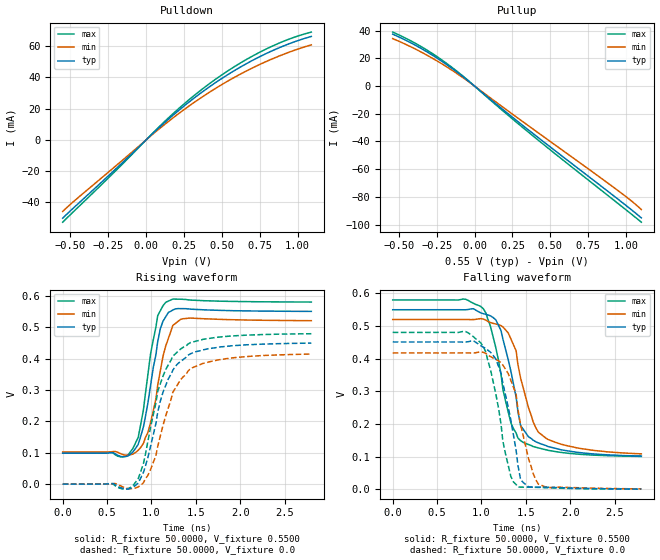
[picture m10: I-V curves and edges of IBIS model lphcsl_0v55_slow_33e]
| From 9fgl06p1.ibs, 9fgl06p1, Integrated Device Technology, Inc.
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[Model]   lphcsl_0v55_slow_33e
Model_type Output
Polarity   Inverting
Enable   Active-High
Vmeas =  0.4000V
Cref =   2.0000pF
Rref =   0.0
Vref =   0.4000V
C_comp   1.1000pF   1.0000pF   1.2000pF
[Temperature Range]   25.0000   85.0000   -40.0
[Voltage Range]   0.5500V   0.5200V   0.5800V
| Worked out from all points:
|   slope of the pulldown table from 0 to 0.083 V, typ, clamps not added: 10.9 ohm
|   slope of the pullup table from 0 to 0.083 V, typ, clamps not added: 10.9 ohm
|   rising waveform, R_fixture 50.0000, V_fixture 0.5500: 20-80 % time 160ps typ, 177ps min, 156ps max; typ from 0.099 V to 0.55 V
|   rising waveform, R_fixture 50.0000, V_fixture 0.0: 20-80 % time 271ps typ, 286ps min, 264ps max; typ from 0 V to 0.449 V
|   falling waveform, R_fixture 50.0000, V_fixture 0.5500: 20-80 % time 210ps typ, 239ps min, 228ps max; typ from 0.55 V to 0.102 V
|   falling waveform, R_fixture 50.0000, V_fixture 0.0: 20-80 % time 190ps typ, 211ps min, 199ps max; typ from 0.451 V to 0.001 V
[Pulldown]
|Voltage   I(typ)   I(min)   I(max)
-550mV    -50.08mA   -45.78mA   -52.65mA
-470mV    -42.74mA   -38.74mA   -45.07mA
-210mV    -19.46mA   -17.46mA   -20.63mA
130mV     11.78mA    10.51mA    12.52mA
250mV     21.68mA    19.4mA     23.02mA
390mV     32.07mA    28.79mA    33.99mA
570mV     43.66mA    39.38mA    46.13mA
750mV     53.32mA    48.34mA    56.16mA
930mV     61.07mA    55.69mA    64.05mA
1.09V     66.25mA    60.88mA    69.05mA
[Pullup]
|Voltage   I(typ)   I(min)   I(max)
-540mV    37.52mA    34.32mA    39.03mA
-440mV    32.37mA    29.43mA    33.82mA
-340mV    26.43mA    23.9mA     27.73mA
-240mV    19.68mA    17.7mA     20.72mA
-140mV    12.09mA    10.82mA    12.77mA
360mV     -32.05mA   -29mA      -33.69mA
920mV     -79.46mA   -73.36mA   -82.52mA
1.02V     -88.05mA   -81.67mA   -91.22mA
1.1V      -95.23mA   -89.17mA   -98.31mA
[Ramp]
| variable   typ   min   max
dV/dt_r  0.2696/0.2691n   0.2487/0.2857n   0.2876/0.2561n
dV/dt_f  0.2689/0.2333n   0.2469/0.2701n   0.2876/0.2220n
R_load = 50.0000
[Rising Waveform]
R_fixture= 50.0000
V_fixture= 0.5500
V_fixture_min= 0.5200
V_fixture_max= 0.5800
|time   V(typ)   V(min)   V(max)
0s        98.56mV    102.4mV    98.79mV
680ps     87.06mV    93.93mV    86.97mV
790ps     101.9mV    95.69mV    113.2mV
850ps     126.6mV    107.7mV    148.9mV
960ps     259.3mV    164.8mV    350.4mV
1.07ns    454.4mV    315.3mV    537.1mV
1.16ns    533.3mV    439.9mV    579.4mV
1.24ns    554.9mV    505.8mV    589.8mV
1.36ns    559.2mV    527.3mV    588.9mV
2.8ns     550.5mV    520.9mV    580.3mV
[Rising Waveform]
R_fixture= 50.0000
V_fixture= 0.0
V_fixture_min= 0.0
V_fixture_max= 0.0
|time   V(typ)   V(min)   V(max)
0s        0V         0V         0V
790ps     -10.68mV   -14.72mV   -5.101mV
910ps     37.96mV    4.791mV    66.39mV
1.05ns    193.4mV    91.13mV    259.1mV
1.07ns    229.3mV    119.9mV    295.8mV
1.13ns    293.2mV    187.7mV    344.4mV
1.24ns    362.9mV    292.5mV    407.7mV
1.44ns    415.6mV    368.5mV    451.3mV
1.89ns    440.5mV    401.6mV    471.9mV
2.8ns     449.4mV    414.5mV    479.3mV
[Falling Waveform]
R_fixture= 50.0000
V_fixture= 0.5500
V_fixture_min= 0.5200
V_fixture_max= 0.5800
|time   V(typ)   V(min)   V(max)
0s        550mV      520mV      580mV
1.02ns    537.8mV    521.5mV    553.2mV
1.1ns     531.5mV    510.9mV    500.2mV
1.22ns    486mV      501.3mV    352.3mV
1.33ns    362.8mV    461.2mV    204.4mV
1.39ns    282.4mV    424.1mV    172.3mV
1.47ns    183.9mV    310.9mV    143.5mV
1.61ns    145.9mV    189.2mV    128.9mV
1.75ns    130.9mV    152.5mV    119.4mV
2.8ns     101.8mV    108.5mV    100.6mV
[Falling Waveform]
R_fixture= 50.0000
V_fixture= 0.0
V_fixture_min= 0.0
V_fixture_max= 0.0
|time   V(typ)   V(min)   V(max)
0s        451.3mV    417.7mV    480.6mV
820ps     451.1mV    417.8mV    483.2mV
990ps     440.2mV    420.8mV    448.9mV
1.1ns     420.3mV    406.7mV    368.3mV
1.22ns    355.3mV    387.7mV    199.7mV
1.33ns    212.2mV    334mV      39.99mV
1.41ns    74.04mV    245.2mV    6.852mV
1.47ns    20.6mV     164mV      6.512mV
1.64ns    6.714mV    15.87mV    5.652mV
2.8ns     737uV      1.275mV    354uV
